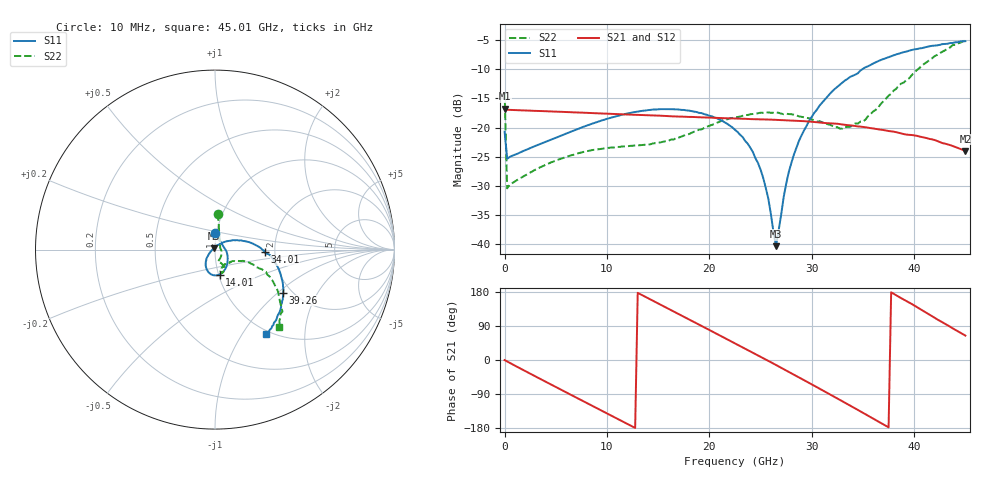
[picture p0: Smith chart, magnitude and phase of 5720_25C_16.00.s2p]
! Device:  ADRF5720
! Description: 0.5dB LSB GaAs MMIC 6-bit Digital Attenuator
! Frequency:  0.000009 -  40 GHz
! Ports:
!	RF1	= Port 1
!	RF2	= Port 2
! Vdd:  3.3 Volt
! Vss:  -3.3 Volt
! Control:  0/3.3 Volt
! State:  16.00 dB attenuation
! Data:  The device was measured using G-S-G Probes on a matrix board.
!  Data was collected using an calibrated 4 port network analyzer.
!  The reference plane for this measurement is at the launchers.
! Note:  Analog Devices supplies this data as a sample of measured data
!  for this product.  Your particular data for this product may vary.
!  Data was taken at 25 degrees C.
!  Analog Devices reserves the right to change this data at anytime.
# GHZ S DB R 45.0
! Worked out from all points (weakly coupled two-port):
!   181 points, 10 MHz to 45.01 GHz, reference 45 ohm
!   highest |S21| = -16.76 dB at 10 MHz (marker M1); lowest = -24.0 dB at 45.01 GHz (marker M2)
!   lowest |S11| = -40.4 dB at 26.51 GHz (marker M3), VSWR 1.02, Z = 44.4 + j0.589 ohm
!   |S11| at or under -10 dB: start of sweep to 34.93 GHz
!   |S22| runs from -30.4 to -5.0 dB; largest |S21 - S12| = 0.00021
!   S11 on the Smith chart (normalised r, x): 10 MHz: 0.98, +0.18; 14.01 GHz: 1.01, -0.29; 34.01 GHz: 1.77, -0.06; 39.26 GHz: 1.81, -1.08; 45.01 GHz: 0.95, -1.28
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0.01  -20.71 90.3  -16.76 -0.2  -16.76 -0.2  -13.95 85.2
0.26  -25.37 8.8  -16.95 -3.9  -16.96 -3.9  -30.44 14.8
4.26  -22.28 -25.4  -17.22 -60.7  -17.22 -60.7  -26.21 -45.4
7.76  -19.84 -47.3  -17.46 -109.6  -17.46 -109.6  -24.17 -67.9
14.01  -17.01 -79.8  -17.89 163.2  -17.90 163.2  -22.90 -73.8
15.26  -16.84 -85.7  -17.97 145.6  -17.98 145.6  -22.54 -70.9
19.26  -17.53 -105.0  -18.25 89.7  -18.25 89.7  -20.31 -63.0
22.76  -20.76 -124.8  -18.47 40.5  -18.47 40.5  -18.20 -65.4
24.01  -23.48 -134.0  -18.55 22.8  -18.55 22.8  -17.71 -67.8
25.01  -27.24 -143.2  -18.58 8.6  -18.58 8.6  -17.45 -69.9
25.76  -32.17 -158.9  -18.63 -2.2  -18.63 -2.2  -17.40 -71.5
26.51  -40.37 136.2  -18.68 -13.0  -18.68 -13.0  -17.42 -73.2
27.26  -31.97 65.0  -18.73 -24.0  -18.74 -24.0  -17.71 -73.7
28.01  -26.11 44.8  -18.81 -34.9  -18.81 -34.8  -17.71 -75.2
28.76  -22.28 36.3  -18.87 -45.8  -18.88 -45.7  -18.09 -75.5
30.26  -17.46 23.2  -19.05 -68.0  -19.05 -68.0  -18.73 -73.5
32.76  -12.65 5.5  -19.42 -105.5  -19.42 -105.4  -20.20 -59.8
34.01  -11.12 -3.0  -19.67 -124.3  -19.68 -124.3  -19.66 -43.4
37.76  -7.74 -24.3  -20.65 178.6  -20.66 178.7  -14.19 -20.5
39.26  -6.96 -32.2  -21.21 155.6  -21.21 155.6  -11.80 -22.8
42.01  -5.94 -45.7  -22.15 111.4  -22.15 111.4  -7.74 -32.5
45.01  -5.17 -59.0  -24.01 64.4  -23.99 64.5  -5.05 -50.1
